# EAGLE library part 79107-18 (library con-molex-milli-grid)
RECEPTACAL
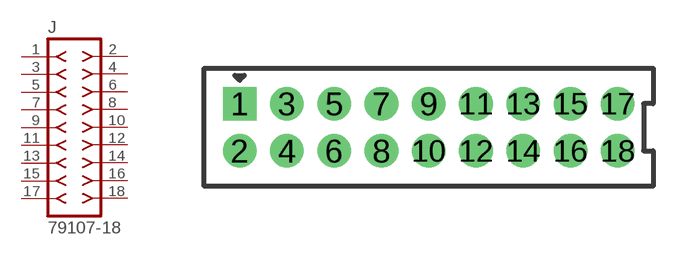
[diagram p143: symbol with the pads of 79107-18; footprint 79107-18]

Designator prefix J

## 79107-18  [79107-18]
1  1  pas
2  2  pas
3  3  pas
4  4  pas
5  5  pas
6  6  pas
7  7  pas
8  8  pas
9  9  pas
10  10  pas
11  11  pas
12  12  pas
13  13  pas
14  14  pas
15  15  pas
16  16  pas
17  17  pas
18  18  pas

## Footprint 79107-18 (pad centres in mm)
RECEPTACAL Dual Row, Vertical, Through-Hole
drill 0.914 square: 1 -8,1
drill 0.914: 2 -8,-1; 3 -6,1; 4 -6,-1; 5 -4,1; 6 -4,-1; 7 -2,1; 8 -2,-1; 9 0,1; 10 0,-1; 11 2,1; 12 2,-1; 13 4,1; 14 4,-1; 15 6,1; 16 6,-1; 17 8,1; 18 8,-1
